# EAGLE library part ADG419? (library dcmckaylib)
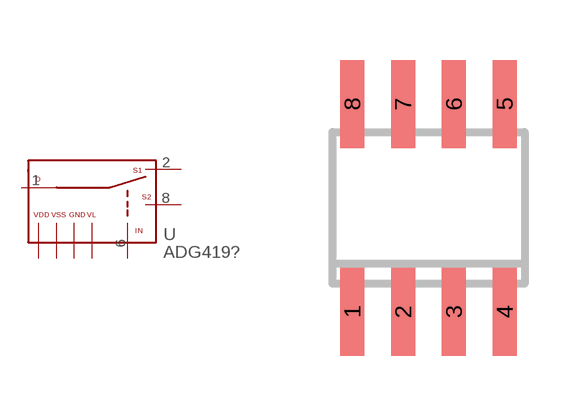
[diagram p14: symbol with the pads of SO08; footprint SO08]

Designator prefix -

## ADG419BR  [SO08]
1  D
2  S1
3  GND  pwr
4  V+  pwr
5  VL  in
6  IN
7  V-  pwr
8  S2

## Footprint SO08 (pad centres in mm)
Small Outline Package 8 NS Package M08A
smd 0.6 x 2.2: 1 -1.905,-2.6; 2 -0.635,-2.6; 3 0.635,-2.6; 4 1.905,-2.6; 5 1.905,2.6; 6 0.635,2.6; 7 -0.635,2.6; 8 -1.905,2.6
